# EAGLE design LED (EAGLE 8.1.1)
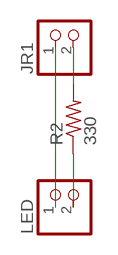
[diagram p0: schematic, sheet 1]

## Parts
JR1  PINHD-1X2  [1X02]
LED  PINHD-1X2  [1X02]
R2  330  R-US_0414/5V  [0414V]

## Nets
N$1: JR1.2 R2.2
N$2: LED.2 R2.1
N$3: JR1.1 LED.1

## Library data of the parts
JR1 LED = pinhead:PINHD-1X2: PIN HEADER
R2 = adafruit:R-US_: RESISTOR, American symbol

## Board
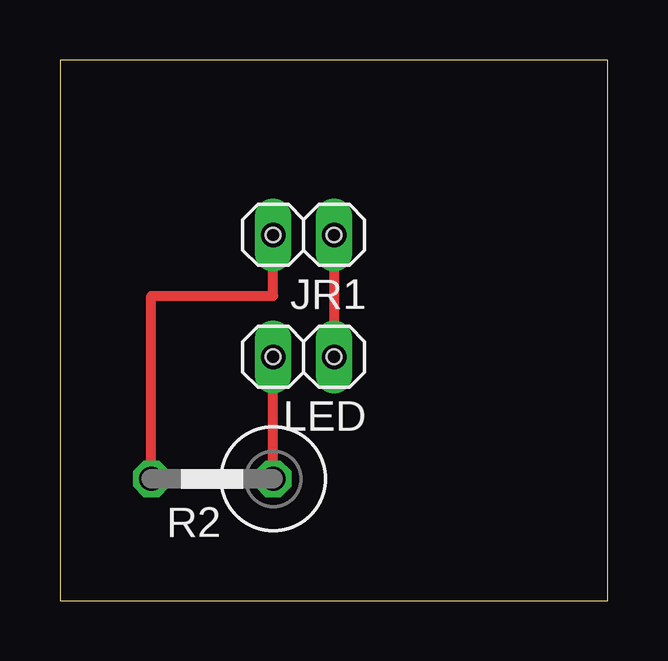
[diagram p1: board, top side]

Size 22.84 x 22.53 mm. Coordinates in mm from the lower left corner, seen from the top.
Outline: 0,0 22.84,0 22.84,22.53 0,22.53 0,0
Copper layers (1*16): Top 0.035mm / dielectric 1.5mm / Bottom 0.035mm
Design rules "default": minimum track width 10mil, minimum drill 24mil, track to track 8mil, track to pad 8mil, pad to pad 8mil, via to via 8mil, smd to smd 8mil, copper to edge 40mil, drill to drill 8mil, minimum pad ring 10mil, minimum via ring 8mil, stop-mask expansion 4mil, vias tented up to drill 0mil, thermal gap 10mil
Holes 0.6 mm at 8.89,15.24 11.43,15.24 8.89,10.16 11.43,10.16 3.81,5.08 8.89,5.08 8.89,15.24

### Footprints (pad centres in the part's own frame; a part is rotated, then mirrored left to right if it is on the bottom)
1X02 = drill 1.016 long: 1 -1.27,0; 2 1.27,0
0414V = drill 1.016 octagon: 1 -2.54,0; 2 2.54,0

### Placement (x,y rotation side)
JR1  10.16,15.24 180 top
LED  10.16,10.16 180 top
R2  6.35,5.08 180 top

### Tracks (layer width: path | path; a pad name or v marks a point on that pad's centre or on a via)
N$1
  Top 0.406: R2.2 3.81,12.7 8.89,12.7 JR1.2
N$2
  Top 0.406: R2.1 LED.2
N$3
  Top 0.406: JR1.1 LED.1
